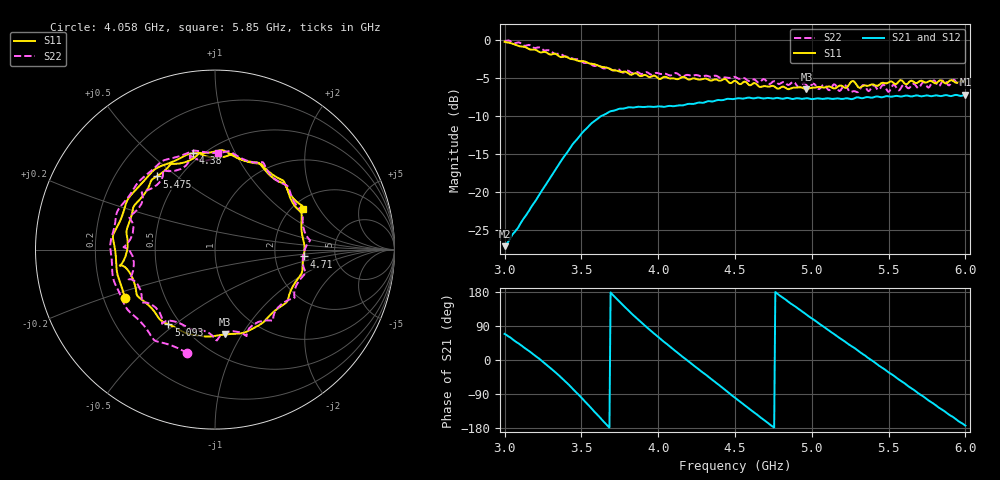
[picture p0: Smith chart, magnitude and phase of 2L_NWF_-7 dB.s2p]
!  26/11/2025  13:44:19
! Ref Plane: 0.000 mm
# MHZ S MA R  50
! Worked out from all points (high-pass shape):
!   401 points, 3 GHz to 6 GHz, reference 50 ohm
!   highest |S21| = -7.18 dB at 6 GHz (marker M1); lowest = -27.1 dB at 3 GHz (marker M2)
!   |S21| within 3 dB of the highest: 3.615 GHz to end of sweep
!   lowest |S11| = -6.4 dB at 4.965 GHz (marker M3), VSWR 2.82, Z = 34.7 - j42.5 ohm
!   |S11| at or under -10 dB: nowhere
!   |S22| runs from -6.8 to 0.0 dB; largest |S21 - S12| = 0.017
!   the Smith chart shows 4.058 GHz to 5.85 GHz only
!   S11 on the Smith chart (normalised r, x): 4.058 GHz: 0.29, -0.23; 4.38 GHz: 0.45, +0.69; 4.71 GHz: 2.93, -0.30; 5.093 GHz: 0.43, -0.47; 5.475 GHz: 0.38, +0.42; 5.85 GHz: 2.27, +1.45
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3000  0.9769 -139.8  0.04422 68.9  0.04428 70.4  0.9883 -105.5
3135  0.9002 -171.4  0.06958 30.4  0.06935 32.1  0.9182 -137.6
3285  0.8136 146.3  0.1191 -16.4  0.1192 -15.0  0.8597 -174.7
3397.5  0.7784 108.3  0.1771 -57.6  0.1774 -56.5  0.781 150.5
3502.5  0.7273 66.6  0.2442 -100.7  0.244 -99.5  0.724 113.7
3622.5  0.6718 17.2  0.3142 -152.5  0.314 -151.3  0.6717 62.7
3735  0.6286 -31.4  0.3507 159.5  0.3502 160.8  0.6472 13.0
3855  0.6059 -79.7  0.3627 112.2  0.3626 113.5  0.6174 -36.4
4005  0.5563 -134.1  0.3671 59.2  0.3667 60.2  0.6037 -89.1
4057.5  0.5689 -151.8  0.3678 41.8  0.3676 43.0  0.5962 -105.0
4177.5  0.5659 169.1  0.3768 2.7  0.3761 4.6  0.5879 -143.3
4380  0.5504 102.9  0.4023 -61.1  0.4035 -59.7  0.5823 157.1
4500  0.5404 63.3  0.4117 -99.4  0.4117 -98.1  0.573 119.6
4710  0.4953 -4.4  0.417 -164.8  0.4148 -164.0  0.5284 56.5
4965  0.4761 -83.2  0.4151 119.8  0.4116 121.0  0.5071 -17.8
5002.5  0.4865 -95.3  0.4097 109.1  0.4062 110.1  0.5137 -30.5
5092.5  0.4911 -121.9  0.4138 83.4  0.411 84.4  0.4963 -52.6
5265  0.5386 -170.4  0.4102 35.1  0.4078 36.3  0.4602 -103.0
5475  0.5214 128.6  0.4259 -24.9  0.423 -23.0  0.5008 -161.5
5505  0.5321 118.7  0.4262 -34.0  0.4246 -32.0  0.4606 -175.5
5850  0.5388 24.9  0.4301 -131.3  0.4293 -129.4  0.537 88.2
6000  0.5334 -17.8  0.4375 -173.2  0.4344 -171.8  0.5357 55.2
